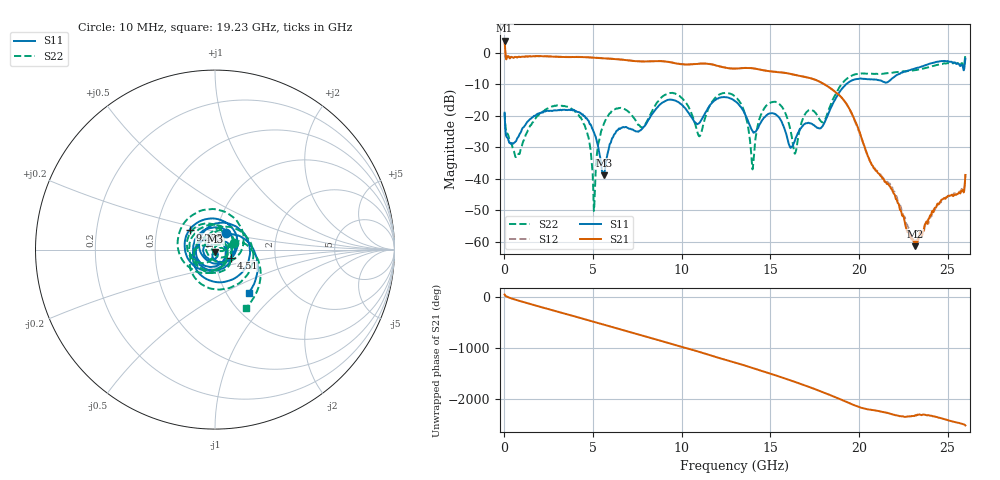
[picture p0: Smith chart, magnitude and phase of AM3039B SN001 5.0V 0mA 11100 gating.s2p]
!Agilent Technologies,E8364B,MY43040894,A.07.50.67
!Agilent E8364B: A.07.50.67
!Date: Tuesday, June 28, 2016 08:12:52
!Correction: S11(Full 2 Port(1,2))
!S21(Full 2 Port(1,2))
!S12(Full 2 Port(1,2))
!S22(Full 2 Port(1,2))
!S2P File: Measurements: S11, S21, S12, S22:
# Hz S  dB  R 50
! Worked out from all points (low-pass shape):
!   1601 points, 10 MHz to 26 GHz, reference 50 ohm
!   highest |S21| = 3.83 dB at 10 MHz (marker M1); lowest = -61.4 dB at 23.14 GHz (marker M2)
!   |S21| within 3 dB of the highest: start of sweep to 43.85 MHz
!   lowest |S11| = -38.9 dB at 5.614 GHz (marker M3), VSWR 1.02, Z = 50.3 - j1.11 ohm
!   |S11| at or under -10 dB: start of sweep to 19.27 GHz
!   |S22| runs from -50.2 to -0.1 dB; largest |S21 - S12| = 0.024
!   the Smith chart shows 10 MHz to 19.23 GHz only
!   S11 on the Smith chart (normalised r, x): 10 MHz: 1.11, +0.21; 4.51 GHz: 1.19, -0.11; 9.285 GHz: 0.74, +0.17; 19.23 GHz: 1.26, -0.68
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1e7  -19.06 56.0  3.83 40.9  3.89 41.7  -19.10 20.6
7.572125e8  -26.92 62.0  -1.38 -73.2  -1.34 -73.0  -32.60 7.6
1.764325e9  -19.89 -23.0  -1.12 -173.6  -1.07 -173.5  -20.77 -48.5
2.852656e9  -18.25 -164.8  -1.27 81.3  -1.22 81.3  -16.80 178.6
4.347081e9  -19.57 -7.5  -1.39 -61.9  -1.36 -61.8  -21.06 -10.9
4.509519e9  -20.09 -27.5  -1.43 -77.7  -1.36 -77.7  -22.87 -31.3
5.045562e9  -25.23 -92.9  -1.57 -130.3  -1.52 -130.3  -50.25 157.2
5.614094e9  -38.89 -76.4  -1.78 174.2  -1.74 174.2  -22.52 8.7
7.319688e9  -24.72 107.8  -2.65 7.4  -2.60 7.4  -20.83 130.1
8.684162e9  -16.97 -133.7  -2.67 -125.6  -2.62 -125.6  -15.35 -142.9
9.285181e9  -14.93 141.9  -2.97 172.4  -2.91 172.3  -12.83 134.4
1.102326e10  -22.10 -159.2  -3.48 1.7  -3.41 1.3  -26.44 -163.0
1.186794e10  -15.09 43.8  -3.94 -89.2  -3.90 -89.5  -14.44 21.9
1.3005e10  -15.33 -105.3  -5.05 157.4  -5.01 156.9  -13.89 -116.2
1.399587e10  -24.84 69.7  -4.94 50.8  -4.91 50.2  -37.05 -156.2
1.601009e10  -28.48 117.8  -6.58 -175.0  -6.56 -175.7  -21.80 53.7
1.734208e10  -22.61 75.6  -8.20 22.4  -8.20 21.6  -18.21 39.7
1.922636e10  -10.26 -52.4  -15.68 121.1  -15.76 119.6  -8.67 -62.4
2.167916e10  -9.07 60.4  -42.07 -111.2  -41.82 -110.8  -6.48 65.5
2.31411e10  -5.04 -57.1  -61.43 -158.3  -59.91 -168.1  -5.53 -49.1
2.47005e10  -2.67 173.0  -46.56 144.9  -46.73 143.4  -3.55 -169.9
2.6e10  -1.86 17.5  -38.81 12.5  -38.56 11.8  -0.12 50.0
